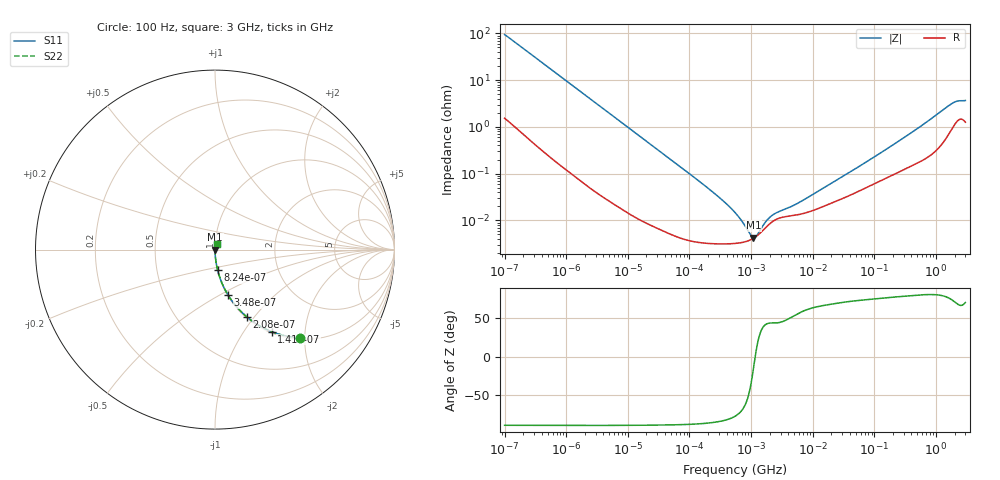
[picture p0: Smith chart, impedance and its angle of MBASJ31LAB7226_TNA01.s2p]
! MBASJ31LAB7226_TNA01  S-PARAMETER MODEL  ( Standard Model )
! Model Generated by TAIYO YUDEN Corporation (http://www.ty-top.com)
! Version 2.0
! TAIYO YUDEN Control No. 230320
! Copyright(c) 2012 TAIYO YUDEN CO.,LTD. All Rights Reserved.
! Product Description (link to TY-COMPAS)
! https://ds.yuden.co.jp/TYCOMPAS/or/detail?pn=MBASJ31LAB7226KTNA01&u=M
! Products Name : Multilayer Ceramic Capacitors
! Characteristics :
!  Capacitance : 22 [uF] , Rated Voltage : 6.3 [V] , TCC : X7R
!  Case Size : 3.2 x 1.6 / 0.126 x 0.063 [mm/inch] , Thickness : 1.6 / 0.063 [mm/inch]
!  (Conditions: Temperature = 25 [degC] , DC Bias Voltage = 0 [V])
! External Node Assignments :
!  1  o---| |---o  2
! GND o---------o GND
! Frequency Range : 100Hz  -  3GHz  [ 401 STEP ]
# MHZ S RI R 50
! Freq[MHz].  S11 Real  S11 Imag  S21 Real  S21 Imag  S12 Real  S12 Imag  S22 Real  S22 Imag
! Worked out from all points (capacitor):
!   401 points, 100 Hz to 3 GHz, reference 50 ohm
!   read as one part in series: C = 16.8 uF near 109 Hz
!   lowest |Z| = 4.3 mohm at 1.091 MHz (marker M1)
!   series resonance near 1.166 MHz, so ESL is about 1.1 nH
!   S11 on the Smith chart (normalised r, x): 100 Hz: 1.03, -1.89; 141 Hz: 1.02, -1.35; 208 Hz: 1.01, -0.92; 348 Hz: 1.01, -0.55; 824 Hz: 1.00, -0.23; 3 GHz: 1.03, +0.07
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0.0001  0.4733 -0.4913  0.5267 0.4913  0.5267 0.4913  0.4733 -0.4913
0.000141  0.315 -0.4569  0.685 0.4569  0.685 0.4569  0.315 -0.4569
0.000208  0.1777 -0.3751  0.8223 0.3751  0.8223 0.3751  0.1777 -0.3751
0.000348  0.0733 -0.2541  0.9267 0.2541  0.9267 0.2541  0.0733 -0.2541
0.000824  0.0149 -0.1152  0.9851 0.1152  0.9851 0.1152  0.0149 -0.1152
0.001788  0.00359 -0.054  0.9964 0.054  0.9964 0.054  0.00359 -0.054
0.005476  0.000556 -0.0179  0.9994 0.0179  0.9994 0.0179  0.000556 -0.0179
0.031977  7.46e-05 -0.0031  0.9999 0.0031  0.9999 0.0031  7.46e-05 -0.0031
0.231582  3.19e-05 -0.000416  1 0.000416  1 0.000416  3.19e-05 -0.000416
0.388167  3.15e-05 -0.000231  1 0.000231  1 0.000231  3.15e-05 -0.000231
0.547723  3.21e-05 -0.000144  1 0.000144  1 0.000144  3.21e-05 -0.000144
0.709116  3.36e-05 -9.03e-05  1 9.03e-05  1 9.03e-05  3.36e-05 -9.03e-05
1.09055  4.14e-05 -1.16e-05  1 1.16e-05  1 1.16e-05  4.14e-05 -1.16e-05
1.75092  7.14e-05 6.4e-05  0.9999 -6.4e-05  0.9999 -6.4e-05  7.14e-05 6.4e-05
2.470636  0.000103 9.73e-05  0.9999 -9.73e-05  0.9999 -9.73e-05  0.000103 9.73e-05
5.135543  0.000129 0.000174  0.9999 -0.000174  0.9999 -0.000174  0.000129 0.000174
9.794414  0.000161 0.000313  0.9998 -0.000313  0.9998 -0.000313  0.000161 0.000313
175.1444  0.000869 0.00356  0.9991 -0.00356  0.9991 -0.00356  0.000869 0.00356
513.708  0.00179 0.00926  0.9982 -0.00926  0.9982 -0.00926  0.00179 0.00926
1789.813  0.00957 0.0294  0.9904 -0.0294  0.9904 -0.0294  0.00957 0.0294
2219.584  0.0142 0.0321  0.9858 -0.0321  0.9858 -0.0321  0.0142 0.0321
3000  0.0136 0.0336  0.9864 -0.0336  0.9864 -0.0336  0.0136 0.0336
